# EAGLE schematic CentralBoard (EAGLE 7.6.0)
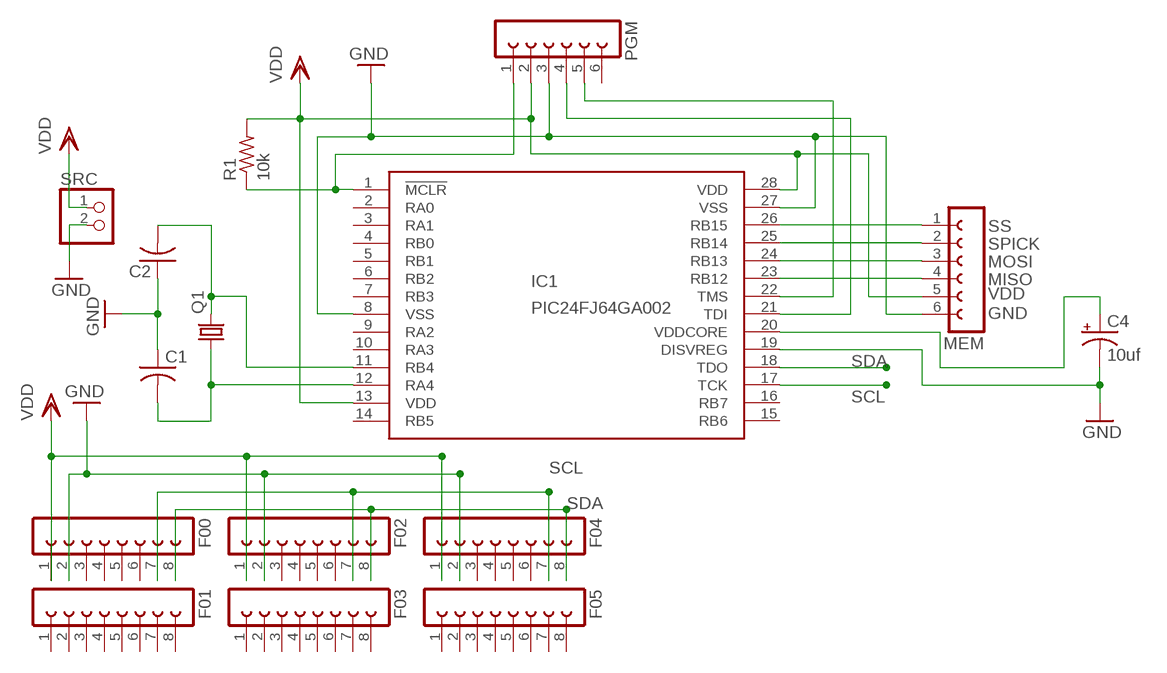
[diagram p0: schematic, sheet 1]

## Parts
C1  C-US025-030X050  [C025-030X050]
C2  C-US025-030X050  [C025-030X050]
C4  10uf  CPOL-USE5-8.5  [E5-8,5]
F00  FE08-1  [FE08]
F01  FE08-1  [FE08]
F02  FE08-1  [FE08]
F03  FE08-1  [FE08]
F04  FE08-1  [FE08]
F05  FE08-1  [FE08]
IC1  PIC24FJ64GA002  [DIL28-3]
MEM  FE06-1  [FE06]
PGM  FE06-1  [FE06]
Q1  CRYSTALTC26V  [TC26V]
R1  10k  R-US_0204/7  [0204/7]
SRC  PINHD-1X2  [1X02]

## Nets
GND: C1.1 C2.1 C4.- F00.2 F02.2 F04.2 IC1.8(VSS) IC1.19(DISVREG) IC1.27(VSS) MEM.6 PGM.3 SRC.2
MISO: IC1.23(RB12) MEM.4
MOSI: IC1.24(RB13) MEM.3
N$1: IC1.1(!MCLR) PGM.1 R1.1
N$2: C1.2 IC1.12(RA4) Q1.1
N$3: C2.2 IC1.11(RB4) Q1.2
N$4: IC1.21(TDI) PGM.4
N$5: IC1.22(TMS) PGM.5
N$6: C4.+ IC1.20(VDDCORE)
SCL: F00.7 F02.7 F04.7 IC1.17(TCK)
SDA: F00.8 F02.8 F04.8 IC1.18(TDO)
SPICK: IC1.25(RB14) MEM.2
SS: IC1.26(RB15) MEM.1
VDD: F00.1 F02.1 F04.1 IC1.13(VDD) IC1.28(VDD) MEM.5 PGM.2 R1.2 SRC.1
Unconnected: F00.3 F00.4 F00.5 F00.6 F01.1 F01.2 F01.3 F01.4 F01.5 F01.6 F01.7 F01.8 F02.3 F02.4 F02.5 F02.6 F03.1 F03.2 F03.3 F03.4 F03.5 F03.6 F03.7 F03.8 F04.3 F04.4 F04.5 F04.6 F05.1 F05.2 F05.3 F05.4 F05.5 F05.6 F05.7 F05.8 IC1.2(RA0) IC1.3(RA1) IC1.4(RB0) IC1.5(RB1) IC1.6(RB2) IC1.7(RB3) IC1.9(RA2) IC1.10(RA3) IC1.14(RB5) IC1.15(RB6) IC1.16(RB7) PGM.6

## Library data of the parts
C1 C2 = adafruit:C-US: CAPACITOR, American symbol
C4 = adafruit:CPOL-US: POLARIZED CAPACITOR, American symbol
F00 F01-F05 = con-lsta:FE08-1: FEMALE HEADER; OC_FARNELL: unknown; OC_NEWARK: unknown
IC1 = microchip:PIC24FJ64GA002: PIC24FJ64GA002 edit this description Auto generated by make-symbol-device-package-bsdl.ulp Rev. 25 Source: PIC24FJ64GA002.bsd; MPN: PIC24FJ64GA002-I/SP; OC_FARNELL: 1332298; OC_NEWARK: 88K6132
MEM PGM = con-lsta:FE06-1: FEMALE HEADER; OC_FARNELL: unknown; OC_NEWARK: unknown
Q1 = crystal:CRYSTAL: CRYSTAL; OC_FARNELL: unknown; OC_NEWARK: unknown
R1 = resistor:R-US_: RESISTOR, American symbol
SRC = pinhead:PINHD-1X2: PIN HEADER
